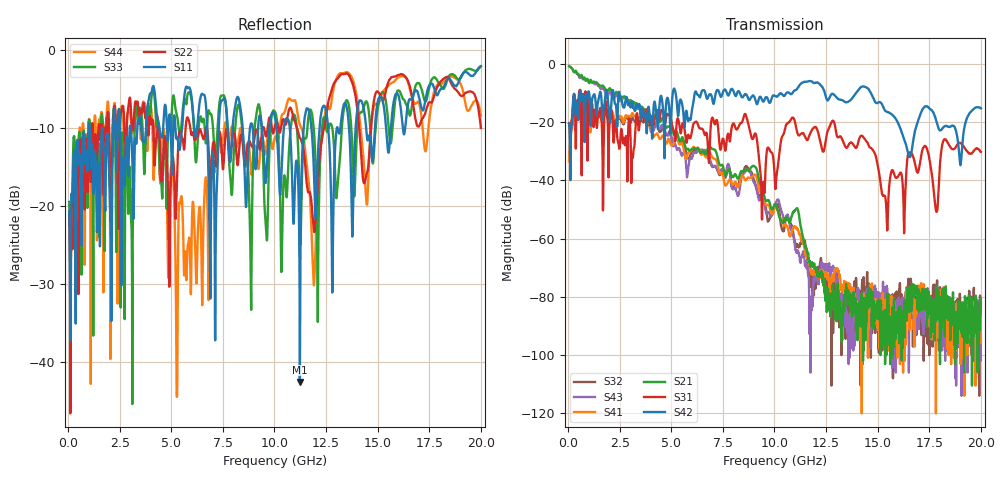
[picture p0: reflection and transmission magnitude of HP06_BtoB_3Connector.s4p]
# MHz S MA R 50.00
! FREQ  S11  S12  S13  S14
!  S21  S22  S23  S24
!  S31  S32  S33  S34
!  S41  S42  S43  S44
!  MAG  ANG  MAG  ANG  MAG  ANG  MAG  ANG
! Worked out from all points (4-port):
!   1996 points, 50 MHz to 20 GHz, reference 50 ohm
!   strongest paths, dB at 50 MHz, 5.04 GHz, 10.03 GHz, 15.02 GHz, 20 GHz:
!     S42: -20.4, -12.4, -10.9, -13.2, -15.2
!     S31: -20.3, -21.0, -42.0, -35.5, -30.2
!     S21: -0.7, -22.5, -48.2, -87.7, -82.2
!     S41: -33.3, -27.8, -49.3, -85.8, -95.9
!     S43: -0.7, -26.9, -48.1, -82.4, -83.1
!     S32: -33.3, -26.8, -49.0, -82.7, -88.2
!   lowest |S11| = -42.6 dB at 11.23 GHz (marker M1), VSWR 1.01, Z = 49.9 + j0.739 ohm
!   |S11| at or under -10 dB: start of sweep to 996.1 MHz; 1.044 GHz to 2.184 GHz (1.14 GHz wide, 70.6 % of centre); 10.74 GHz to 11.42 GHz (677 MHz wide, 6.11 % of centre)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
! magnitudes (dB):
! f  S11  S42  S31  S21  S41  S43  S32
! 50 MHz  -20.7  -20.4  -20.3  -0.7  -33.3  -0.7  -33.3
! 3.79 GHz  -9.5  -21.6  -15.6  -16.2  -20.1  -18.4  -18.9
! 5.26 GHz  -11.4  -12.6  -20.1  -23.3  -24.4  -29.2  -24.5
! 9.45 GHz  -12.0  -12.9  -40.8  -43.7  -45.5  -45.6  -44.1
! 11.23 GHz  -42.6  -7.1  -24.3  -54.0  -58.6  -67.5  -62.3
! 15.43 GHz  -10.9  -16.4  -51.4  -94.0  -82.3  -77.9  -82.0
! 20 GHz  -2.1  -15.2  -30.2  -82.2  -95.9  -83.1  -88.2
